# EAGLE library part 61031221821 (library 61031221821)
Headers & Wire Housings WR-PHD 2.54 mm Dual SMT Socket Header T&R Source: Datasheet
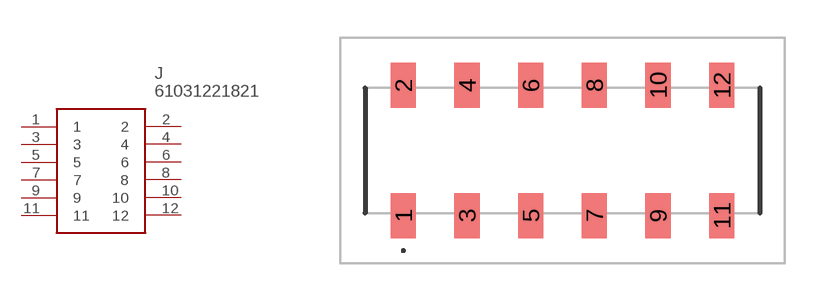
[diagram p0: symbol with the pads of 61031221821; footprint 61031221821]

Designator prefix J

## 61031221821 (Description: Headers & Wire Housings WR-PHD 2.54 mm Dual SMT Socket Header T&R; Height: 7.75mm; Manufacturer_Name: Wurth Elektronik; Manufacturer_Part_Number: 61031221821; Mouser_Part_Number: 710-61031221821; Mouser_Price-Stock: https://www.mouser.co.uk/ProductDetail/Wurth-Elektronik/61031221821?qs=Cb2nCFKsA8qsJuA9v2g26A%3D%3D)  [61031221821]
1  1
2  2
3  3
4  4
5  5
6  6
7  7
8  8
9  9
10  10
11  11
12  12

## Footprint 61031221821 (pad centres in mm)
61031221821-1
smd 1 x 1.8: 1 -6.35,-2.6; 2 -6.35,2.6; 3 -3.81,-2.6; 4 -3.81,2.6; 5 -1.27,-2.6; 6 -1.27,2.6; 7 1.27,-2.6; 8 1.27,2.6; 9 3.81,-2.6; 10 3.81,2.6; 11 6.35,-2.6; 12 6.35,2.6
